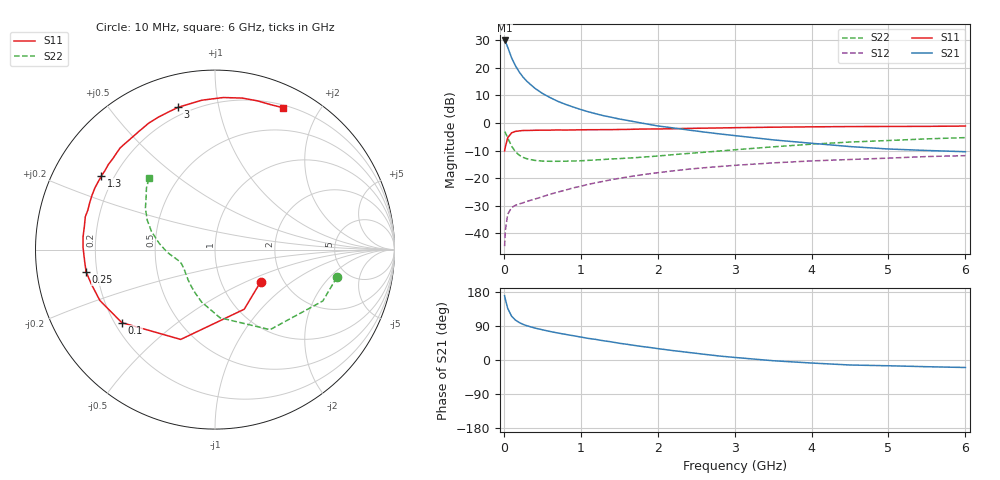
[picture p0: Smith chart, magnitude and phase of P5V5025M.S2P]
! SIEMENS Small Signal Semiconductors
! BFP183
! Si NPN RF Bipolar Junction Transistor in SOT143
! VCE = 0.5 V  IC = 25 mA
! Common Emitter S-Parameters:  March  1996
# GHz  S  MA  R  50
!  f  S11  S21  S12  S22
! GHz  MAG  ANG  MAG  ANG  MAG  ANG  MAG  ANG
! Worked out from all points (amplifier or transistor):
!   36 points, 10 MHz to 6 GHz, reference 50 ohm
!   highest |S21| = 29.8 dB at 10 MHz (marker M1)
!   |S21| within 3 dB of that: start of sweep to 57.51 MHz
!   unconditionally stable (mu >= 1): start of sweep to 13.62 MHz; 264.1 MHz to end of sweep
!   at 250 MHz: K = 0.96, MSG = 22.7 dB, |S12| = -28.9 dB
!   at 1.4 GHz: K = 1.87, MAG = 5.9 dB, |S12| = -20.5 dB
!   at 6 GHz: K = 1.50, MAG = -3.5 dB, |S12| = -11.8 dB
!   S11 on the Smith chart (normalised r, x): 10 MHz: 1.54, -0.61; 100 MHz: 0.23, -0.33; 250 MHz: 0.16, -0.08; 1.3 GHz: 0.15, +0.29; 3 GHz: 0.16, +0.76; 6 GHz: 0.23, +1.56
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0.01  0.3113 -35.2  30.92 169.6  0.0059 73.5  0.6958 -12.9
0.02  0.37 -63.9  29.62 159.9  0.0114 70.3  0.6653 -25.5
0.05  0.5357 -110.9  23.38 136.4  0.0223 51.6  0.5414 -55.5
0.1  0.6597 -141.9  15.09 115.9  0.0293 37.7  0.3808 -85.8
0.15  0.7014 -156.2  10.83 105.4  0.0324 33.8  0.3015 -104.3
0.2  0.7158 -164.6  8.331 98.9  0.0342 33.8  0.2607 -116.4
0.25  0.7287 -170.2  6.718 94.0  0.0359 34.2  0.2381 -125.4
0.3  0.729 -174.5  5.644 90.4  0.0381 36.2  0.2241 -132.4
0.4  0.7349 179.3  4.266 84.5  0.0418 39.8  0.21 -141.3
0.5  0.7386 174.2  3.414 79.8  0.0461 42.3  0.2039 -147.2
0.6  0.7391 170.0  2.872 75.3  0.0512 45.1  0.2022 -151.8
0.7  0.7455 165.8  2.458 71.3  0.056 46.6  0.2021 -155.0
0.9  0.7454 159.5  1.939 64.2  0.0667 48.6  0.2044 -158.8
1.1  0.7523 152.9  1.585 57.0  0.0776 49.4  0.21 -162.3
1.3  0.7543 147.1  1.346 50.6  0.0881 49.0  0.218 -165.2
1.7  0.7679 135.7  1.047 38.4  0.1101 46.7  0.234 -170.0
2.2  0.7835 122.6  0.811 24.8  0.1356 42.1  0.2663 -177.0
3  0.8189 104.5  0.589 6.8  0.1706 33.1  0.326 170.9
3.5  0.8355 95.1  0.493 -1.9  0.1891 27.7  0.3689 163.9
4.5  0.8578 79.8  0.373 -13.2  0.2177 16.9  0.4504 149.4
5.5  0.8652 69.0  0.317 -17.7  0.246 7.7  0.5139 138.0
6  0.8761 64.5  0.301 -19.8  0.2556 2.7  0.5416 132.7
